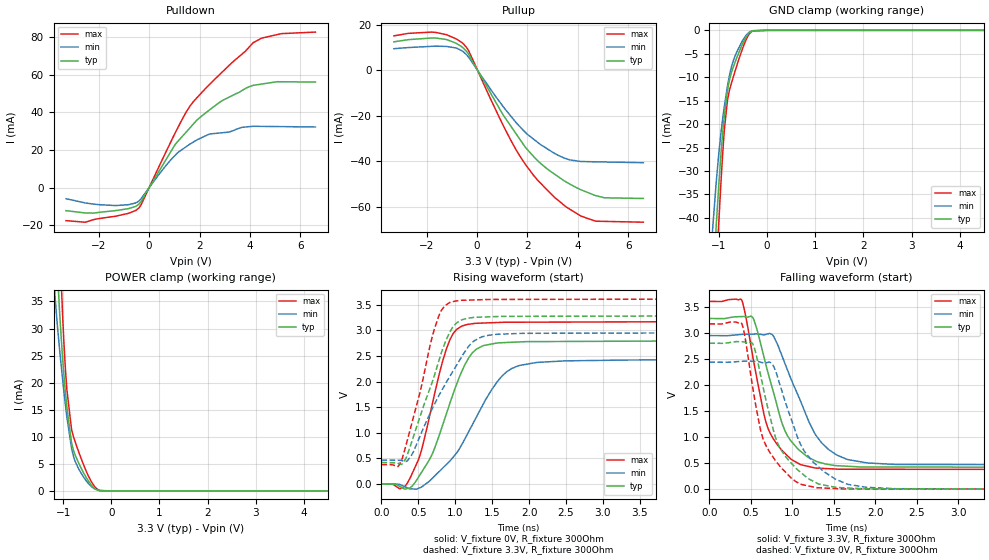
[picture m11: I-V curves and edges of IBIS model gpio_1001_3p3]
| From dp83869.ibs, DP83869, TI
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|   gpio_1001_3p3 Model
[Model]   gpio_1001_3p3
Model_type   I/O
Polarity   Non-Inverting
Enable   Active-Low
Vinl = 0.7
Vinh = 1.7
Vmeas = 1.65
Vref = 0
Cref = 2pF
Rref = 100000
|   typ   min   max
C_comp   1.10585pF   1.10585pF   1.45739pF
| Where Nom  PVT is Nominal Process, 3.3V,  27C
|   Fast PVT is Strong Process,  3.63V, -40C
|   Slow PVT is Weak Process,   2.97V, 125C
[Voltage Range]   3.3   2.97   3.63
|Junction Temperature
[Temperature Range]   27   125   -40
[Pullup Reference]   3.3   2.97   3.63
[Pulldown Reference]   -0   -0   0
[Power Clamp Reference]   3.3   2.97   3.63
[GND Clamp Reference]   0   0   0
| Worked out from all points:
|   slope of the pulldown table from 0 to 0.495 V, typ, clamps not added: 45 ohm
|   slope of the pullup table from 0 to 0.495 V, typ, clamps not added: 51.7 ohm
|   GND clamp passes 1 mA (typ) near -0.41 V on its own axis
|   POWER clamp passes 1 mA (typ) near -0.41 V on its own axis
|   falling waveform, V_fixture 3.3V, R_fixture 300Ohm: 20-80 % time 324ps typ, 416ps min, 271ps max; typ from 3.28 V to 0.421 V
|   rising waveform, V_fixture 0V, R_fixture 300Ohm: 20-80 % time 422ps typ, 593ps min, 322ps max; typ from 0 V to 2.8 V
|   rising waveform, V_fixture 3.3V, R_fixture 300Ohm: 20-80 % time 400ps typ, 544ps min, 323ps max; typ from 0.421 V to 3.28 V
|   falling waveform, V_fixture 0V, R_fixture 300Ohm: 20-80 % time 343ps typ, 413ps min, 292ps max; typ from 2.81 V to 0 V
[Pulldown]
|   Voltage   I(typ)   I(min)   I(max)
-3.3V     -12.23mA   -5.88mA    -17.54mA
-2.521V   -13.46mA   -8.179mA   -18.32mA
-1.331V   -12.2mA    -9.541mA   -15.19mA
-507.9mV  -9.779mA   -7.981mA   -11.91mA
-302.9mV  -6.968mA   -5.579mA   -8.646mA
889.4mV   19.76mA    15.18mA    25.08mA
1.49V     29.76mA    21.88mA    40.51mA
2.52V     42.49mA    28.6mA     56.41mA
3.852V    52.81mA    32.18mA    72.84mA
4.467V    54.94mA    32.48mA    79.3mA
5.249V    56.15mA    32.36mA    81.69mA
6.6V      55.99mA    32.15mA    82.51mA
[GND Clamp]
|   Voltage   I(typ)   I(min)   I(max)
-3.3V     -489.2mA   -422.2mA   -556.8mA
-1.128V   -53.94mA   -41.75mA   -66.49mA
-1.053V   -40.94mA   -31.89mA   -50.85mA
-1.004V   -32.91mA   -26.23mA   -40.88mA
-914.8mV  -20.88mA   -18.15mA   -24.96mA
-886mV    -17.91mA   -16.01mA   -20.9mA
-824.7mV  -12.98mA   -11.96mA   -14.96mA
-737.5mV  -8.884mA   -7.637mA   -11.14mA
-632.6mV  -5.898mA   -4.664mA   -7.616mA
-450.4mV  -1.653mA   -1.242mA   -2.33mA
-360.4mV  -415.6uA   -340.7uA   -627.7uA
6.6V      0A         0A         0A
[Pullup]
|   Voltage   I(typ)   I(min)   I(max)
-3.3V     12.49mA    9.464mA    15.12mA
-1.707V   14.15mA    10.54mA    16.68mA
-1.212V   13.5mA     10.46mA    15.6mA
-593mV    10.22mA    8.516mA    12.07mA
-324.7mV  6.819mA    5.568mA    8.362mA
899.7mV   -17.05mA   -13.91mA   -21.09mA
1.626V    -29.13mA   -23.9mA    -36.35mA
2.293V    -38.43mA   -30.68mA   -46.82mA
3.057V    -45.46mA   -36.36mA   -55.63mA
3.682V    -49.97mA   -39.36mA   -61.01mA
4.705V    -55.02mA   -40.19mA   -66.27mA
6.6V      -56.29mA   -40.59mA   -66.7mA
[POWER Clamp]
|   Voltage   I(typ)   I(min)   I(max)
-3.3V     592.7mA    473.7mA    711.1mA
-1.183V   53.33mA    37.6mA     74.54mA
-1.164V   49.45mA    35.35mA    69.48mA
-1.121V   40.99mA    30.62mA    58.01mA
-1.071V   32.56mA    25.84mA    45.66mA
-1.013V   24.62mA    20.7mA     32.69mA
-952.4mV  18.17mA    15.83mA    22.43mA
-922.7mV  15.44mA    13.63mA    18.69mA
-824.7mV  8.834mA    7.855mA    11.3mA
-669.2mV  4.995mA    3.928mA    7.01mA
-332.6mV  387.6uA    312.9uA    668.4uA
6.6V      0A         0A         0A
[Ramp]
R_load = 300
|   typ   min   max
dV/dt_r   1.67961/4.19848e-10   1.45816/5.89428e-10   1.90434/3.20143e-10
dV/dt_f   1.71823/3.234e-10   1.49249/4.14197e-10   1.94043/2.70728e-10
[Falling Waveform]
V_fixture = 3.3V
V_fixture_min = 2.97V
V_fixture_max = 3.63V
R_fixture = 300Ohm
C_fixture = 0F
|   Time   V(typ)   V(min)   V(max)
0s        3.284V     2.955V     3.613V
388.9ps   3.321V     2.978V     3.641V
525ps     3.299V     2.984V     2.536V
709.4ps   2.226V     2.989V     1.161V
773.6ps   1.859V     2.942V     963.4mV
910.2ps   1.129V     2.423V     691.4mV
1.092ns   739.3mV    1.724V     478.3mV
1.352ns   505.5mV    894.3mV    400.8mV
1.681ns   439.7mV    566mV      383.6mV
5ns       420.6mV    467.7mV    379mV
[Rising Waveform]
V_fixture = 0V
V_fixture_min = 0V
V_fixture_max = 0V
R_fixture = 300Ohm
C_fixture = 0F
|   Time   V(typ)   V(min)   V(max)
0s        212.8uV    321uV      218.6uV
254.6ps   -52.51mV   -11.92mV   -91.68mV
385.8ps   -75.59mV   -95mV      109.8mV
548.8ps   240.9mV    -53.95mV   694.7mV
877.6ps   1.362V     378.5mV    2.628V
1.083ns   2.181V     757.4mV    3.08V
1.363ns   2.693V     1.518V     3.144V
1.644ns   2.761V     2.125V     3.159V
1.872ns   2.776V     2.316V     3.161V
5ns       2.8V       2.431V     3.174V
[Rising Waveform]
V_fixture = 3.3V
V_fixture_min = 2.97V
V_fixture_max = 3.63V
R_fixture = 300Ohm
C_fixture = 0F
|   Time   V(typ)   V(min)   V(max)
0s        420.6mV    467.7mV    379mV
219.8ps   405.6mV    463.1mV    339.7mV
272.8ps   383.2mV    457.9mV    467.5mV
396.4ps   763.1mV    534.5mV    1.104V
718.1ps   2.125V     1.556V     3.031V
812.6ps   2.567V     1.817V     3.393V
918.5ps   2.945V     2.084V     3.54V
1.22ns    3.248V     2.753V     3.594V
1.452ns   3.266V     2.906V     3.604V
5ns       3.284V     2.955V     3.613V
[Falling Waveform]
|Gnd
V_fixture = 0V
V_fixture_min = 0V
V_fixture_max = 0V
R_fixture = 300Ohm
C_fixture = 0F
|   Time   V(typ)   V(min)   V(max)
0s        2.809V     2.443V     3.18V
388.9ps   2.836V     2.459V     3.191V
433.9ps   2.826V     2.464V     2.888V
519.1ps   2.807V     2.46V      1.992V
630.1ps   2.098V     2.438V     1.057V
796.7ps   995.8mV    2.28V      551mV
1.106ns   317.2mV    843.6mV    94.74mV
1.518ns   36.92mV    195.2mV    12.03mV
1.895ns   6.88mV     35.68mV    5.082mV
5ns       206.2uV    304.3uV    214.6uV
